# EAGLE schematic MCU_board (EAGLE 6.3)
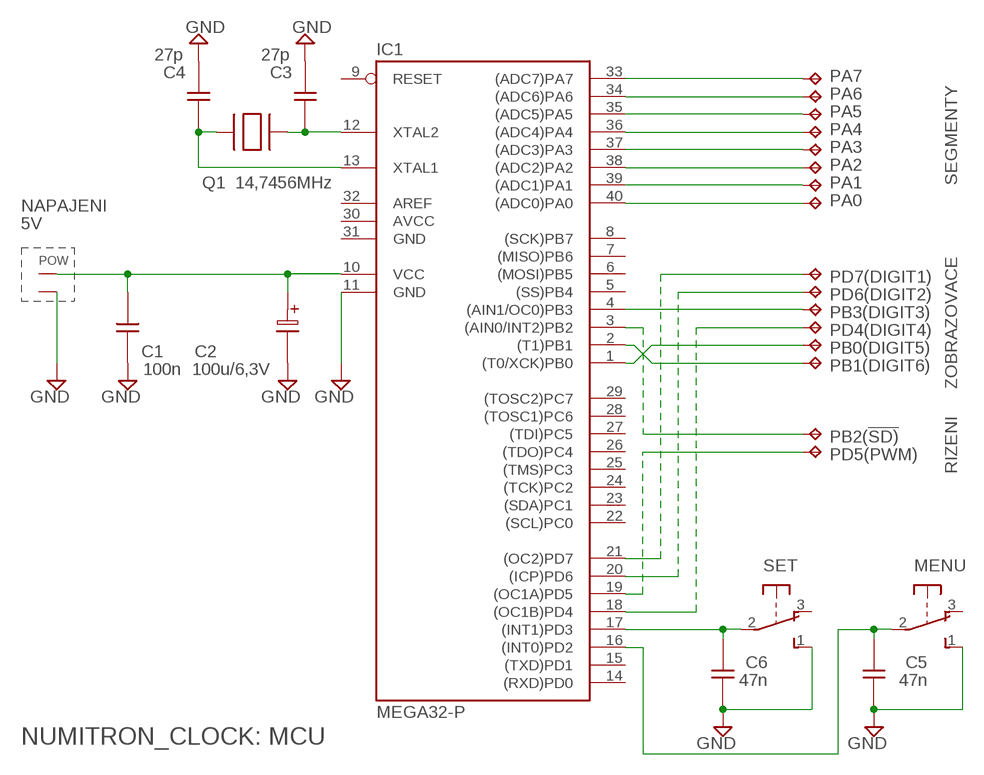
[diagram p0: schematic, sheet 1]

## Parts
C1  100n  CK  [CK]
C2  100u/6,3V  CT15  [CT15]
C3  27p  CK  [CK]
C4  27p  CK  [CK]
C5  47n  CK  [CK]
C6  47n  CK  [CK]
IC1  MEGA32-P  [DIL40]
MENU  9077-1  [9077-1]
PA0  TPPAD1-13Y  [P1-13Y]
PA1  TPPAD1-13Y  [P1-13Y]
PA2  TPPAD1-13Y  [P1-13Y]
PA3  TPPAD1-13Y  [P1-13Y]
PA4  TPPAD1-13Y  [P1-13Y]
PA5  TPPAD1-13Y  [P1-13Y]
PA6  TPPAD1-13Y  [P1-13Y]
PA7  TPPAD1-13Y  [P1-13Y]
PB0(DIGIT5)  TPPAD1-13Y  [P1-13Y]
PB1(DIGIT6)  TPPAD1-13Y  [P1-13Y]
PB2(!SD)  TPPAD1-13Y  [P1-13Y]
PB3(DIGIT3)  TPPAD1-13Y  [P1-13Y]
PD4(DIGIT4)  TPPAD1-13Y  [P1-13Y]
PD5(PWM)  TPPAD1-13Y  [P1-13Y]
PD6(DIGIT2)  TPPAD1-13Y  [P1-13Y]
PD7(DIGIT1)  TPPAD1-13Y  [P1-13Y]
POW  ARK500/2  [ARK500/2]
Q1  14,7456MHz  QHC-18  [HC-18]
SET  9077-1  [9077-1]

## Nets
GND: C1.1 C2.2 C3.1 C4.1 C5.1 C6.1 IC1.11(GND) MENU.1(S) POW.2 SET.1(S)
N$1: C3.2 IC1.12(XTAL2) Q1.1
N$2: IC1.4((AIN1/OC0)PB3) PB3(DIGIT3).TP
N$3: C4.2 IC1.13(XTAL1) Q1.2
N$4: IC1.2((T1)PB1) PB1(DIGIT6).TP
N$5: C5.2 IC1.16((INT0)PD2) MENU.2(P)
N$6: IC1.33((ADC7)PA7) PA7.TP
N$7: IC1.34((ADC6)PA6) PA6.TP
N$8: IC1.35((ADC5)PA5) PA5.TP
N$9: IC1.36((ADC4)PA4) PA4.TP
N$10: IC1.37((ADC3)PA3) PA3.TP
N$11: IC1.38((ADC2)PA2) PA2.TP
N$12: IC1.39((ADC1)PA1) PA1.TP
N$13: IC1.40((ADC0)PA0) PA0.TP
N$14: IC1.1((T0/XCK)PB0) PB0(DIGIT5).TP
N$15: IC1.21((OC2)PD7) PD7(DIGIT1).TP
N$16: IC1.20((ICP)PD6) PD6(DIGIT2).TP
N$17: IC1.18((OC1B)PD4) PD4(DIGIT4).TP
N$18: IC1.19((OC1A)PD5) PD5(PWM).TP
N$19: IC1.3((AIN0/INT2)PB2) PB2(!SD).TP
N$20: C6.2 IC1.17((INT1)PD3) SET.2(P)
V+: C1.2 C2.1 IC1.10(VCC) POW.1
Unconnected: IC1.5((SS)PB4) IC1.6((MOSI)PB5) IC1.7((MISO)PB6) IC1.8((SCK)PB7) IC1.9(RESET) IC1.14((RXD)PD0) IC1.15((TXD)PD1) IC1.22((SCL)PC0) IC1.23((SDA)PC1) IC1.24((TCK)PC2) IC1.25((TMS)PC3) IC1.26((TDO)PC4) IC1.27((TDI)PC5) IC1.28((TOSC1)PC6) IC1.29((TOSC2)PC7) IC1.32(AREF) MENU.3(O) SET.3(O)

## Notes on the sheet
- SEGMENTY
- NAPAJENI
- 5V
- ZOBRAZOVACE
- RIZENI
- NUMITRON_CLOCK: MCU

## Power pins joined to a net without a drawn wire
AVCC: IC1.30(AVCC)
GND: IC1.31(GND)

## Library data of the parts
C1 C3-C6 = #_GM99:CK
C2 = #_GM99:CT15: RM = 5mm, R = 10mm
IC1 = atmel:MEGA32-P: MICROCONTROLLER 32 Kbytes FLASH 2 Kbytes SRAM 1 Kbytes EEPROM USART 8-channel 10 bit ADC Source: www.atmel.com .. doc2503.pdf; MPN: ATMEGA32-16PU; OC_FARNELL: 1661729; OC_NEWARK: 51P1794
MENU SET = switch-misc:9077-1: MARQUARDT SWITCH 9077.0100 Distributor: Buerklin
PA0 PA1-PA7 PB0(DIGIT5) PB1(DIGIT6) PB2(!SD) PB3(DIGIT3) PD4(DIGIT4) PD5(PWM) PD6(DIGIT2) PD7(DIGIT1) = testpad:TP: Test pad
POW = #_GM99:ARK500/2
Q1 = #_GM99:QHC-18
